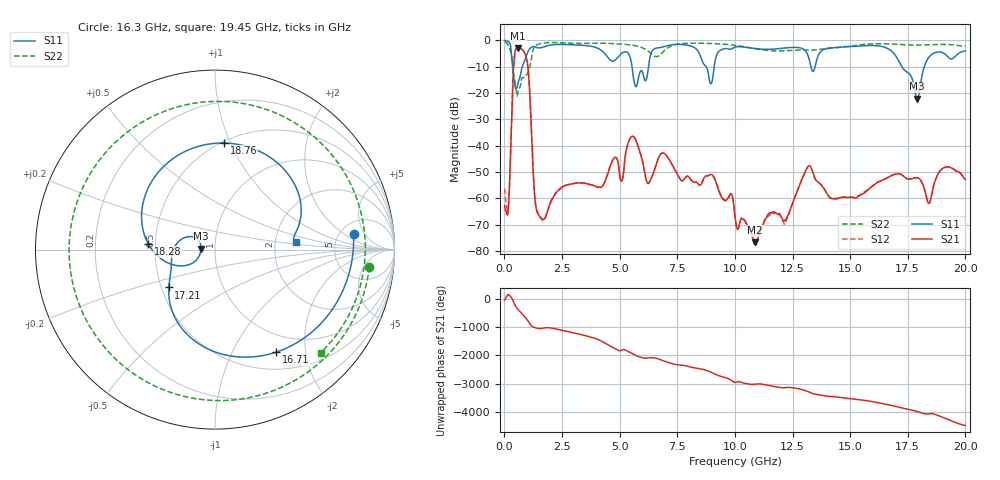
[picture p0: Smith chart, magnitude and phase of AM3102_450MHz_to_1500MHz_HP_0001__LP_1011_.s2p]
!Agilent Technologies,E8364B,MY43040894,A.07.50.67
!Agilent E8364B: A.07.50.67
!Date: Thursday, January 11, 2018 05:22:15
!Correction: S11(Full 2 Port(1,2))
!S21(Full 2 Port(1,2))
!S12(Full 2 Port(1,2))
!S22(Full 2 Port(1,2))
!S2P File: Measurements: S11, S21, S12, S22:
# Hz S  dB  R 50
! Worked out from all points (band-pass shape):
!   1601 points, 10 MHz to 20 GHz, reference 50 ohm
!   highest |S21| = -2.89 dB at 597.2 MHz (marker M1); lowest = -76.7 dB at 10.88 GHz (marker M2)
!   |S21| within 3 dB of the highest: 438.1 MHz to 924.7 MHz (486.6 MHz wide, 71.4 % of centre)
!   lowest |S11| = -22.2 dB at 17.91 GHz (marker M3), VSWR 1.17, Z = 42.8 + j0.408 ohm
!   |S11| at or under -10 dB: 356.4 MHz to 775.4 MHz (419 MHz wide, 74 % of centre); 5.538 GHz to 6.251 GHz (712.7 MHz wide, 12.1 % of centre); 17.24 GHz to 18.22 GHz (971.8 MHz wide, 5.48 % of centre)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
!   |S22| runs from -21.1 to -0.5 dB; largest |S21 - S12| = 0.002
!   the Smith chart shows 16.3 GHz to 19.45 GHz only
!   S11 on the Smith chart (normalised r, x): 16.3 GHz: 6.67, +2.91; 16.71 GHz: 0.73, -1.50; 17.21 GHz: 0.55, -0.26; 18.28 GHz: 0.46, +0.03; 18.76 GHz: 0.52, +0.95; 19.45 GHz: 2.61, +0.27
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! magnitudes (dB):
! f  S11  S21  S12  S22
! 10 MHz  0.0  -62.6  -56.3  -0.5
! 172.4 MHz  -0.6  -63.2  -62.9  -2.1
! 409.8 MHz  -14.4  -8.7  -8.7  -13.1
! 597.2 MHz  -16.0  -2.9  -2.9  -19.4
! 997 MHz  -4.8  -8.6  -8.6  -12.6
! 1.484 GHz  -2.9  -66.4  -66.0  -1.4
! 3.346 GHz  -1.9  -54.1  -54.2  -1.2
! 5.707 GHz  -17.6  -37.9  -38.0  -2.1
! 6.682 GHz  -2.8  -44.7  -44.7  -6.0
! 8.956 GHz  -16.5  -50.9  -51.0  -1.2
! 10.01 GHz  -2.6  -66.7  -67.2  -1.9
! 10.88 GHz  -3.1  -76.7  -77.9  -3.2
! 13.34 GHz  -11.3  -49.1  -49.0  -3.7
! 16.3 GHz  -2.2  -53.5  -53.3  -1.3
! 16.68 GHz  -3.3  -51.9  -51.9  -1.3
! 16.71 GHz  -3.5  -51.7  -51.7  -1.3
! 17.21 GHz  -9.6  -50.8  -50.9  -1.6
! 17.91 GHz  -22.2  -52.2  -52.1  -1.8
! 18.28 GHz  -8.6  -58.2  -58.1  -1.7
! 18.76 GHz  -4.5  -51.6  -51.6  -1.6
! 19.45 GHz  -6.9  -48.8  -48.6  -1.7
! 20 GHz  -4.0  -52.9  -52.9  -2.3
